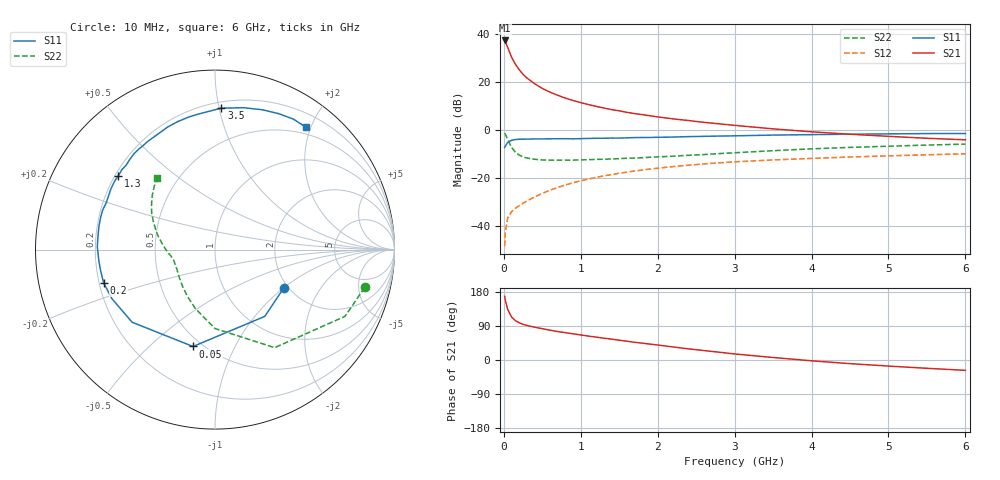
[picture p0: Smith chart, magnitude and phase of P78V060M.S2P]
! SIEMENS Small Signal Semiconductors
! BFP196
! Si NPN RF Bipolar Junction Transistor in SOT143
! VCE = 8 V  IC = 60 mA
! Common Emitter S-Parameters:  May  1996
# GHz  S  MA  R  50
!  f  S11  S21  S12  S22
! GHz  MAG  ANG  MAG  ANG  MAG  ANG  MAG  ANG
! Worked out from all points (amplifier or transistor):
!   36 points, 10 MHz to 6 GHz, reference 50 ohm
!   highest |S21| = 37.4 dB at 10 MHz (marker M1)
!   |S21| within 3 dB of that: start of sweep to 51.07 MHz
!   unconditionally stable (mu >= 1): 470.4 MHz to 4.5 GHz
!   at 250 MHz: K = 0.82, MSG = 26.9 dB, |S12| = -30.5 dB
!   at 1.4 GHz: K = 1.08, MAG = 11.8 dB, |S12| = -18.5 dB
!   at 6 GHz: K = 0.98, MSG = 2.9 dB, |S12| = -9.9 dB
!   S11 on the Smith chart (normalised r, x): 10 MHz: 1.90, -1.00; 50 MHz: 0.45, -0.70; 200 MHz: 0.22, -0.14; 1.3 GHz: 0.21, +0.33; 3.5 GHz: 0.24, +1.02; 6 GHz: 0.39, +1.92
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0.01  0.4388 -28.9  74.3 168.2  0.0038 79.9  0.8603 -14.2
0.02  0.4641 -53.3  69.11 156.9  0.0076 71.1  0.8141 -27.2
0.05  0.5536 -102.8  53.12 133.6  0.0147 55.1  0.6395 -58.7
0.1  0.6141 -138.8  33.56 113.7  0.0199 47.5  0.4392 -90.1
0.15  0.6361 -154.6  23.64 104.0  0.0235 47.9  0.3473 -108.2
0.2  0.6475 -163.3  18.19 98.2  0.0267 50.1  0.3023 -120.6
0.25  0.648 -169.8  14.6 94.1  0.03 53.0  0.2763 -130.0
0.3  0.6502 -174.3  12.27 91.2  0.0333 55.6  0.2627 -136.3
0.4  0.6559 178.6  9.29 86.5  0.0406 58.3  0.2468 -146.0
0.5  0.6564 173.3  7.42 82.6  0.0479 60.5  0.2392 -152.3
0.6  0.6596 168.5  6.207 78.7  0.056 61.3  0.237 -156.7
0.7  0.6619 164.1  5.335 75.1  0.0636 61.4  0.2367 -160.0
0.9  0.6598 156.5  4.155 69.1  0.0799 60.6  0.2371 -165.0
1.1  0.6717 149.6  3.414 63.1  0.0956 59.2  0.2426 -168.3
1.3  0.6779 142.5  2.893 57.5  0.1112 56.8  0.2476 -171.6
1.7  0.6994 130.2  2.216 46.7  0.1406 51.7  0.2619 -177.1
2.2  0.7173 116.6  1.719 34.5  0.1737 44.4  0.2862 176.3
2.8  0.7527 101.3  1.354 20.6  0.208 35.8  0.3247 166.8
3.5  0.7891 87.4  1.064 6.6  0.2391 25.8  0.3726 156.5
4.5  0.8229 71.2  0.821 -9.6  0.2751 14.1  0.4367 144.1
5.5  0.8481 59.0  0.677 -21.9  0.3064 3.5  0.4886 133.9
6  0.8494 53.5  0.629 -27.3  0.3206 -2.1  0.5121 129.0
